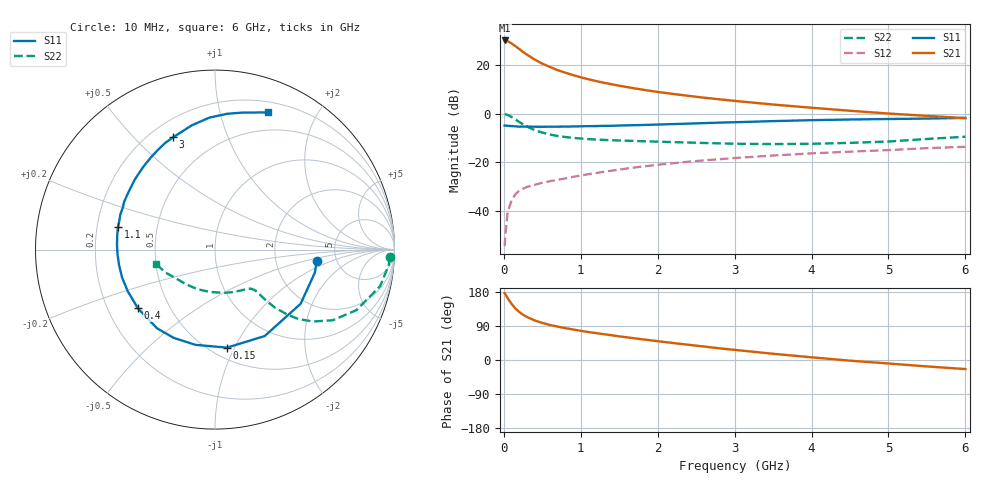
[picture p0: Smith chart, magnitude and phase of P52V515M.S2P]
! SIEMENS Small Signal Semiconductors
! BFP183
! Si NPN RF Bipolar Junction Transistor in SOT143
! VCE = 2.5 V  IC = 15 mA
! Common Emitter S-Parameters:  March  1996
# GHz  S  MA  R  50
!  f  S11  S21  S12  S22
! GHz  MAG  ANG  MAG  ANG  MAG  ANG  MAG  ANG
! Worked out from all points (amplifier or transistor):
!   36 points, 10 MHz to 6 GHz, reference 50 ohm
!   highest |S21| = 30.1 dB at 10 MHz (marker M1)
!   |S21| within 3 dB of that: start of sweep to 178.4 MHz
!   unconditionally stable (mu >= 1): 929.3 MHz to 5.598 GHz
!   at 250 MHz: K = 0.42, MSG = 28.1 dB, |S12| = -30.8 dB
!   at 1.4 GHz: K = 1.13, MAG = 15.6 dB, |S12| = -23.4 dB
!   at 6 GHz: K = 0.94, MSG = 5.9 dB, |S12| = -13.6 dB
!   S11 on the Smith chart (normalised r, x): 10 MHz: 3.51, -0.67; 150 MHz: 0.60, -0.93; 400 MHz: 0.33, -0.30; 1.1 GHz: 0.29, +0.10; 3 GHz: 0.29, +0.65; 6 GHz: 0.30, +1.41
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0.01  0.5701 -6.5  31.95 176.6  0.0019 88.4  0.9767 -2.5
0.02  0.5711 -12.9  31.84 173.4  0.0033 82.5  0.9716 -5.1
0.05  0.5646 -32.3  30.96 163.0  0.0095 77.9  0.9423 -12.5
0.1  0.5555 -60.1  27.82 148.3  0.0164 65.7  0.8578 -23.1
0.15  0.5502 -83.0  24.44 136.1  0.0222 57.8  0.7646 -31.0
0.2  0.5416 -101.6  21.32 126.7  0.0262 53.3  0.6768 -36.3
0.25  0.543 -115.1  18.51 119.3  0.0288 49.6  0.6035 -39.8
0.3  0.5446 -126.4  16.35 113.7  0.0313 48.0  0.5447 -41.9
0.4  0.5398 -142.7  12.99 104.4  0.0345 46.2  0.4627 -44.1
0.5  0.5388 -154.5  10.66 97.8  0.0381 45.0  0.4092 -44.8
0.6  0.5407 -163.4  9.107 92.4  0.041 46.1  0.373 -45.1
0.7  0.5415 -171.1  7.834 88.0  0.0439 46.7  0.3484 -45.1
0.8  0.5437 -177.2  6.944 84.0  0.0468 47.4  0.3316 -45.2
1  0.5503 171.9  5.587 77.0  0.0537 49.0  0.3089 -46.1
1.1  0.555 167.1  5.106 73.7  0.0572 49.1  0.3006 -46.8
1.5  0.5716 152.5  3.757 62.4  0.0711 49.7  0.2817 -51.1
2.2  0.6113 130.4  2.544 44.8  0.0961 46.6  0.2607 -63.6
3  0.6675 110.5  1.833 26.7  0.1229 40.9  0.2414 -83.3
3.5  0.7039 100.7  1.543 16.4  0.1383 36.8  0.2377 -97.8
4.5  0.7598 84.9  1.149 -1.8  0.1661 28.4  0.2516 -129.5
5.5  0.7945 74.0  0.902 -17.0  0.196 20.9  0.3027 -154.8
6  0.8186 69.0  0.811 -23.9  0.2088 16.2  0.3366 -165.9
